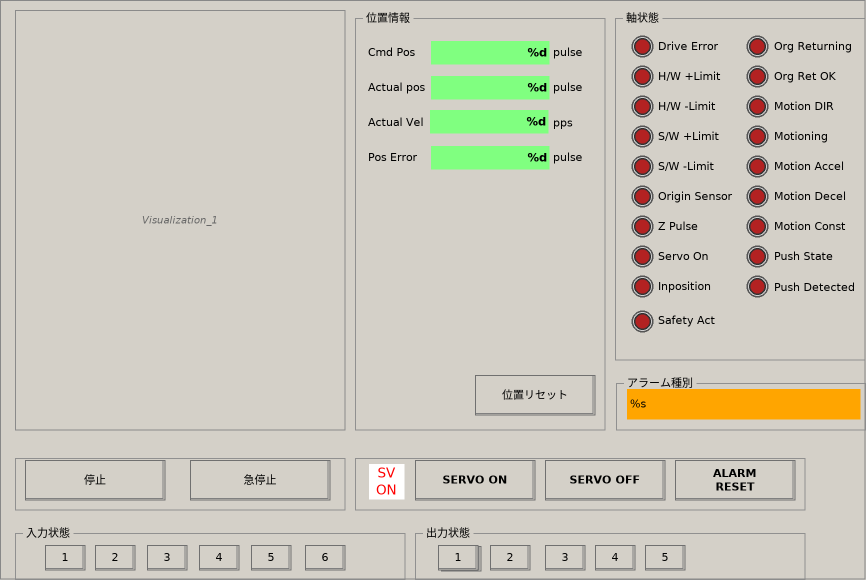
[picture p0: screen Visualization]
VISUALIZATION Visualization  // 866x580
    GroupBox (355,10 250x420), "位置情報"
        Button (120,365 120x40), "位置リセット"
            tap main.pos_reset
        Label (10,30 60x25), "Cmd Pos"
        Label (10,65 60x25), "Actual pos"
        Label (10,100 60x25), "Actual Vel"
        Label (10,135 60x25), "Pos Error"
        Label (195,30 40x25), "pulse"
        Label (195,65 40x25), "pulse"
        Label (195,100 40x26), "pps"
        Label (195,135 40x25), "pulse"
        Textfield (75,30 120x25), "%d", text variable: main.cmd_pos_count
        Textfield (75,65 120x25), "%d", text variable: main.act_pos_count
        Textfield (74,99 120x25), "%d", text variable: main.actual_vel
        Textfield (75,135 120x25), "%d", text variable: main.pos_error_count
    GroupBox (615,10 250x350), "軸状態"
        Lamp1 (15,24 25x25), variable: main.drive_error, style: Lamp-Lamp1-Red
        Lamp1 (15,54 25x25), variable: main.lim_p, style: Lamp-Lamp1-Red
        Lamp1 (15,84 25x25), variable: main.lim_m, style: Lamp-Lamp1-Red
        Lamp1 (15,114 25x25), variable: main.sw_p_limit, style: Lamp-Lamp1-Red
        Lamp1 (15,144 25x25), style: Lamp-Lamp1-Red
        Lamp1 (15,174 25x25), variable: main.org, style: Lamp-Lamp1-Red
        Lamp1 (15,204 25x25), variable: main.z_pulse, style: Lamp-Lamp1-Red
        Lamp1 (15,234 25x25), variable: main.enable_ope, style: Lamp-Lamp1-Red
        Lamp1 (15,264 25x25), variable: main.inposition, style: Lamp-Lamp1-Red
        Lamp1 (15,299 25x25), variable: main.Safty_act_led, style: Lamp-Lamp1-Red
        Lamp1 (130,54 25x25), variable: main.org_ret_led, style: Lamp-Lamp1-Red
        Lamp1 (130,24 25x25), variable: main.org_returning_led, style: Lamp-Lamp1-Red
        Lamp1 (130,84 25x25), variable: main.motion_dir_led, style: Lamp-Lamp1-Red
        Lamp1 (130,114 25x25), variable: main.motioning_led, style: Lamp-Lamp1-Red
        Lamp1 (130,144 25x25), variable: main.motion_accel_led, style: Lamp-Lamp1-Red
        Lamp1 (130,174 25x25), variable: main.motion_decel_led, style: Lamp-Lamp1-Red
        Lamp1 (130,204 25x25), variable: main.motion_const_led, style: Lamp-Lamp1-Red
        Lamp1 (130,234 25x25), variable: main.push_state_led, style: Lamp-Lamp1-Red
        Lamp1 (130,264 25x25), variable: main.push_detected_led, style: Lamp-Lamp1-Red
        Label (156,24 85x25), "Org Returning"
        Label (40,174 85x25), "Origin Sensor"
        Label (40,298 85x25), "Safety Act"
        Label (40,264 85x25), "Inposition"
        Label (40,234 85x25), "Servo On"
        Label (40,204 85x25), "Z Pulse"
        Label (40,144 85x25), "S/W -Limit"
        Label (40,114 85x25), "S/W +Limit"
        Label (40,84 85x25), "H/W -Limit"
        Label (40,54 85x25), "H/W +Limit"
        Label (40,24 85x25), "Drive Error"
        Label (156,84 85x25), "Motion DIR"
        Label (156,114 85x25), "Motioning"
        Label (156,144 85x25), "Motion Accel"
        Label (156,174 85x25), "Motion Decel"
        Label (156,204 85x25), "Motion Const"
        Label (156,234 85x25), "Push State"
        Label (156,265 85x25), "Push Detected"
        Label (156,54 85x25), "Org Ret OK"
    GroupBox (15,450 330x60)
        Button (10,10 140x40), "停止"
            tap main.stop_dec
        Button (175,10 140x40), "急停止"
            tap main.stop_imm
    GroupBox (355,450 450x60)
        Button (60,10 120x40), "SERVO ON"
            tap main.enable_on
        Button (190,10 120x40), "SERVO OFF"
            tap main.enable_off
        Button (320,10 120x40), "ALARM RESET"
            tap main.alarm_reset_sw
        Rectangle (14,14 35x35), "SV OFF", invisible if: main.enable_ope
        Rectangle (14,14 35x35), "SV ON", invisible if: main.enable_ope_n
    GroupBox (616,375 250x55), "アラーム種別"
        Textfield (11,14 233x30), "%s", text variable: error_code.alarm_type, invisible if: error_code.err
    GroupBox (15,525 390x55), "入力状態"
        Rectangle (583,22 35x20), "5"
        Button (30,20 40x25), "1", colour toggle: main.in1
        Button (80,20 40x25), "2", colour toggle: main.in2
        Button (290,20 40x25), "6", colour toggle: main.in6
        Button (236,20 40x25), "5", colour toggle: main.in5
        Button (184,20 40x25), "4", colour toggle: main.in4
        Button (132,20 40x25), "3", colour toggle: main.in3
        Button (426,21 40x25), "1", colour toggle: main.in1
    GroupBox (415,525 390x55), "出力状態"
        Button (23,20 40x25), "1", colour toggle: main.out1
            OnMouseClick: toggle main.out1
        Button (75,20 40x25), "2", colour toggle: main.out2
            OnMouseClick: toggle main.out2
        Button (130,20 40x25), "3", colour toggle: main.out3
            OnMouseClick: toggle main.out3
        Button (180,20 40x25), "4", colour toggle: main.out4
            OnMouseClick: toggle main.out4
        Button (230,20 40x25), "5", colour toggle: main.out5
            OnMouseClick: toggle main.out5
    TabControl (15,10 330x420), frame switch variable: main.mode_of_ope
        shows Visualization_1()
        shows Visualization_2()
        shows Visualization_3()
        [0]: TabTitle=一般動作
        [1]: TabTitle=原点復帰
        [2]: TabTitle=Push動作
END_VISUALIZATION
